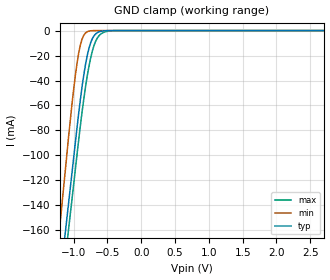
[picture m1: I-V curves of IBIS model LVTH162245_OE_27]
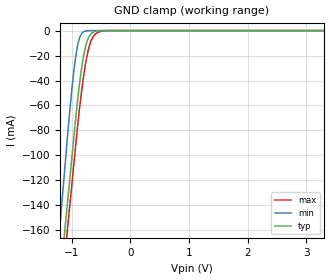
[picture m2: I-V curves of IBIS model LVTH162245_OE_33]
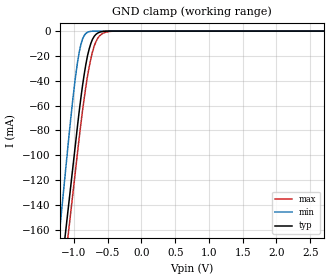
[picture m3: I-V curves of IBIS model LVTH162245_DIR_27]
| TEXAS INSTRUMENTS INCORPORATED
| Standard Linear and Logic Group
| IBIS Model of SN54LVTH162245
| 3.3-V ABT 16-BIT BUS TRANSCEIVERS WITH 3-STATE OUTPUTS
| This file contains package information for the following:
|  SOIC 48-pin (WD) package as [Component] LVTH162245_WD
| This device can be powered at the following Vccs:
|  2.7 volt Vcc
|  3.3 volt Vcc
| This file provides unique models under the [Model Selector] for each Vcc.
| For operation at a specific Vcc, select the appropriate model after each
| [Model Selector] keyword.
[IBIS Ver]   3.2
[Comment char]  |_char
[File Name]   sn54lvth162245.ibs
[File Rev]   1.1 | b_die
[Date]   March 27, 2003
[Source]   Data created from TI-SPICE simulations at TI-SLL.
[Notes]   The following is an IBIS list for the LVTH162245.
   Please contact sllibis@ti.com with questions and
   comments concerning SLL IBIS models.
   - Power-clamp data has been deleted since there is no
   power-clamp diode in the device.
   - Due to presence of bus hold at input, GND-clamp curves
   have non-monotonic warnings.
   - Non-monotonic data in pullup/pulldown data due to damping
   resistor.
[Disclaimer] Property of Texas Instruments Incorporated.  Unauthorized
   reproduction and/or distribution is strictly prohibited.
   This product is protected under copyright law.
   Created  2003, (C) Copyright  2003, Texas Instruments
   Incorporated, All Rights Reserved
   UNLESS THERE IS A SIGNED, WRITTEN AGREEMENT TO THE
   CONTRARY, TEXAS INSTRUMENTS (TI) IS PROVIDING THE IBIS
   MODELS  AND WITHOUT ANY WARRANTY, EXPRESSED OR
   IMPLIED.  TI assumes no liability for:
   1) the accuracy of the IBIS models provided to your
   company;
   2) the proper functioning of these IBIS Models in your
   design or for any resulting applications; or
   3) infringement of patents, copyrights or intellectual
   property rights resulting from your use of these IBIS
   models.
   TI provides IBIS Models as a service to our customers.
   You and your company shall not distribute, sell or give
   these models to anyone else without prior written
   permission from TI.
   TI reserves the right to make changes to our products or
   to discontinue any semiconductor product or service
   without notice, and advises our customers to obtain the
   latest version of relevant information to verify, before
   placing orders, that the information being relied on is
   current.
   Please be aware that your receipt and use of the IBIS
   information provided shall serve as acceptance of these
   terms and conditions.  If you do not accept these terms,
   you should return or destroy the IBIS models and any
   other accompanying information immediately.
| Component LVTH162245_WD 48-pin SOIC
[Component]   LVTH162245_WD
[Manufacturer]   Texas Instruments, Inc.
[Package]
|   typ   min   max
R_pkg   0.161   0.116   0.231
L_pkg   6.816e-9   4.867e-9   10.108e-9
C_pkg   2.468e-12   1.62e-12   3.698e-12
[Pin]   signal_name   model_name   R_pin   L_pin   C_pin
1   1DIR   LVTH162245_DIR   0.231   10.108e-9   3.220e-12
2   1B1   LVTH162245_BIO   0.224   9.570e-9   3.698e-12
3   1B2   LVTH162245_BIO   0.202   8.681e-9   3.350e-12
4   GND   GND   0.185   7.877e-9   2.960e-12
5   1B3   LVTH162245_BIO   0.170   7.118e-9   2.404e-12
6   1B4   LVTH162245_BIO   0.155   6.481e-9   2.131e-12
7   VCC   POWER   0.138   5.760e-9   2.150e-12
8   1B5   LVTH162245_BIO   0.135   5.641e-9   2.103e-12
9   1B6   LVTH162245_BIO   0.134   5.593e-9   2.070e-12
10   GND   GND   0.120   5.070e-9   1.812e-12
11   1B7   LVTH162245_BIO   0.119   5.022e-9   1.793e-12
12   1B8   LVTH162245_BIO   0.116   4.868e-9   1.651e-12
13   2B1   LVTH162245_BIO   0.116   4.867e-9   1.658e-12
14   2B2   LVTH162245_BIO   0.119   5.024e-9   1.805e-12
15   GND   GND   0.121   5.074e-9   1.825e-12
16   2B3   LVTH162245_BIO   0.134   5.595e-9   2.105e-12
17   2B4   LVTH162245_BIO   0.136   5.644e-9   2.144e-12
18   VCC   POWER   0.139   5.763e-9   2.197e-12
19   2B5   LVTH162245_BIO   0.155   6.483e-9   2.152e-12
20   2B6   LVTH162245_BIO   0.157   6.535e-9   2.172e-12
21   GND   GND   0.164   6.944e-9   2.459e-12
22   2B7   LVTH162245_BIO   0.174   7.397e-9   2.657e-12
23   2B8   LVTH162245_BIO   0.189   7.964e-9   2.834e-12
24   2DIR   LVTH162245_DIR   0.188   8.149e-9   2.455e-12
25   2NOE   LVTH162245_OE   0.188   8.148e-9   2.455e-12
26   2A8   LVTH162245_AIO   0.189   7.963e-9   2.834e-12
27   2A7   LVTH162245_AIO   0.174   7.396e-9   2.658e-12
28   GND   GND   0.164   6.943e-9   2.461e-12
29   2A6   LVTH162245_AIO   0.157   6.535e-9   2.174e-12
30   2A5   LVTH162245_AIO   0.168   7.064e-9   2.384e-12
31   VCC   POWER   0.159   6.694e-9   2.687e-12
32   2A4   LVTH162245_AIO   0.163   6.925e-9   2.828e-12
33   2A3   LVTH162245_AIO   0.169   7.198e-9   2.967e-12
34   GND   GND   0.163   7.027e-9   2.887e-12
35   2A2   LVTH162245_AIO   0.162   6.977e-9   2.868e-12
36   2A1   LVTH162245_AIO   0.167   7.207e-9   2.815e-12
37   1A8   LVTH162245_AIO   0.149   6.371e-9   2.557e-12
38   1A7   LVTH162245_AIO   0.139   5.942e-9   2.312e-12
39   GND   GND   0.149   6.375e-9   2.428e-12
40   1A6   LVTH162245_AIO   0.135   5.649e-9   2.135e-12
41   1A5   LVTH162245_AIO   0.137   5.708e-9   2.174e-12
42   VCC   POWER   0.129   5.341e-9   1.804e-12
43   1A4   LVTH162245_AIO   0.124   5.115e-9   1.620e-12
44   1A3   LVTH162245_AIO   0.170   7.117e-9   2.402e-12
45   GND   GND   0.185   7.876e-9   2.956e-12
46   1A2   LVTH162245_AIO   0.202   8.680e-9   3.347e-12
47   1A1   LVTH162245_AIO   0.224   9.570e-9   3.696e-12
48   1NOE   LVTH162245_OE   0.231   10.108e-9   3.219e-12
| Model LVTH162245_OE
[Model Selector]   LVTH162245_OE
LVTH162245_OE_27   2.7 volt Vcc
LVTH162245_OE_33   3.3 volt Vcc
| Model LVTH162245_DIR
[Model Selector]   LVTH162245_DIR
LVTH162245_DIR_27   2.7 volt Vcc
LVTH162245_DIR_33   3.3 volt Vcc
| Model LVTH162245_AIO
[Model Selector]   LVTH162245_AIO
LVTH162245_AIO_27   2.7 volt Vcc
LVTH162245_AIO_33   3.3 volt Vcc
| Model LVTH162245_BIO
[Model Selector]   LVTH162245_BIO
LVTH162245_BIO_27   2.7 volt Vcc
LVTH162245_BIO_33   3.3 volt Vcc
| Models and submodels in the file (8): LVTH162245_OE_27 (Input), LVTH162245_OE_33 (Input), LVTH162245_DIR_27 (Input), LVTH162245_DIR_33 (Input), LVTH162245_AIO_27 (I/O), LVTH162245_AIO_33 (I/O), LVTH162245_BIO_27 (I/O), LVTH162245_BIO_33 (I/O)
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[Model]   LVTH162245_OE_27
Model_type  Input
Vinl = 0.8
Vinh = 2.0
| variable   typ   min   max
C_comp   3.58pF   2.76pF   4.61pF
[Temperature Range]   40   -40   100
| Ambient temperature   25   -40   85
[Voltage range]   2.7   2.7   2.7
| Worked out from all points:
|   GND clamp passes 1 mA (typ) near -0.62 V on its own axis
[GND Clamp]
| LVTH162245_OE_27
|   Voltage   I(typ)   I(min)   I(max)
-5.5V     -2.288A    -2.547A    -2.284A
-1.225V   -210.8mA   -168.1mA   -231.1mA
-1.195V   -196.3mA   -151.5mA   -216.7mA
-1.135V   -167.2mA   -118.2mA   -187.9mA
-1.105V   -152.7mA   -101.6mA   -173.6mA
-1.075V   -138.1mA   -84.99mA   -159.2mA
-975mV    -89.73mA   -35.97mA   -111.2mA
-900mV    -54.95mA   -11.36mA   -75.86mA
-775mV    -14.49mA   -458.2uA   -29.04mA
-700mV    -4.229mA   -21.87uA   -12.08mA
-600mV    -595.8uA   -186.1nA   -2.835mA
2.7V      9.09pA     2.798pA    676.8pA
[Model]   LVTH162245_OE_33
Model_type  Input
Vinl = 0.8
Vinh = 2.0
| variable   typ   min   max
C_comp   3.55pF   2.61pF   4.44pF
[Temperature Range]   40   -40   100
| Ambient temperature   25   -40   85
[Voltage range]   3.3   3   3.6
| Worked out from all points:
|   GND clamp passes 1 mA (typ) near -0.62 V on its own axis
[GND Clamp]
| LVTH162245_OE_33
|   Voltage   I(typ)   I(min)   I(max)
-5.5V     -2.288A    -2.547A    -2.284A
-1.225V   -210.8mA   -168.1mA   -231.1mA
-1.195V   -196.3mA   -151.5mA   -216.7mA
-1.135V   -167.2mA   -118.2mA   -187.9mA
-1.105V   -152.7mA   -101.6mA   -173.6mA
-1.075V   -138.1mA   -84.99mA   -159.2mA
-975mV    -89.73mA   -35.97mA   -111.2mA
-900mV    -54.95mA   -11.36mA   -75.86mA
-775mV    -14.49mA   -458.2uA   -29.04mA
-700mV    -4.229mA   -21.87uA   -12.08mA
-600mV    -595.8uA   -186.1nA   -2.835mA
3.3V      11.11pA    3.42pA     1.265nA
[Model]   LVTH162245_DIR_27
Model_type  Input
Vinl = 0.8
Vinh = 2.0
| variable   typ   min   max
C_comp   3.57pF   2.74pF   4.59pF
[Temperature Range]   40   -40   100
| Ambient temperature   25   -40   85
[Voltage range]   2.7   2.7   2.7
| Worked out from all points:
|   GND clamp passes 1 mA (typ) near -0.62 V on its own axis
[GND Clamp]
| LVTH162245_DIR_27
|   Voltage   I(typ)   I(min)   I(max)
-5.5V     -2.288A    -2.547A    -2.284A
-1.225V   -210.8mA   -168.1mA   -231.1mA
-1.195V   -196.3mA   -151.5mA   -216.7mA
-1.135V   -167.2mA   -118.2mA   -187.9mA
-1.105V   -152.7mA   -101.6mA   -173.6mA
-1.075V   -138.1mA   -84.99mA   -159.2mA
-975mV    -89.73mA   -35.97mA   -111.2mA
-900mV    -54.95mA   -11.36mA   -75.86mA
-775mV    -14.49mA   -458.2uA   -29.04mA
-700mV    -4.229mA   -21.87uA   -12.08mA
-600mV    -595.8uA   -186.1nA   -2.835mA
2.7V      9.09pA     2.798pA    676.8pA
